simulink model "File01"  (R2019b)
settings: Solver=FixedStepDiscrete  StartTime=0.0  StopTime=20  FixedStep=1  RelTol=1e-3
libraries: simulink x1

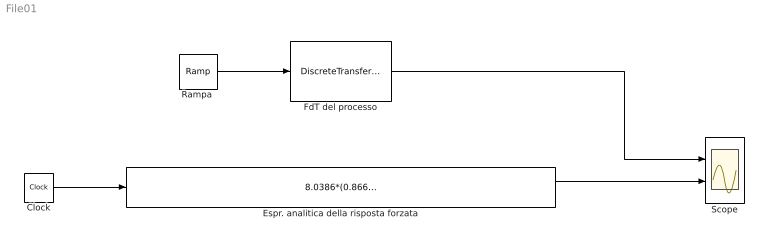
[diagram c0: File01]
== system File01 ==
  Clock : Clock
  Espr. analitica della risposta forzata : Fcn  Expr=8.0386*(0.866)^u-0.0415*(-0.866)^u-8+0.9998*u
  FdT del processo : DiscreteTransferFcn  Denominator=[4 0 -3]
  "Rampa " : simulink/Sources/Ramp  slope=1  start=0  InitialOutput=0
  Scope : Scope  NumInputPorts=2
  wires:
  "Rampa "/1 -> FdT del processo/1
  Clock/1 -> Espr. analitica della risposta forzata/1
  FdT del processo/1 -> Scope/1
  Espr. analitica della risposta forzata/1 -> Scope/2
